FUNCTION_BLOCK FB_SignalHandlingDelay EXTENDS FB_SignalHandling
VAR_INPUT
	tDelay				: TIME;			// 延迟时间
END_VAR
VAR
	bStartProcessing	: BOOL;			// 开始延迟
	fbTimerDelay		: TON;			// TON功能块
END_VAR

// =========================================================
;
// =========================================================

METHOD SetOutput
VAR_INPUT
END_VAR
// =========================================================

IF bEnableLocal AND bInput THEN
	bStartProcessing := TRUE;
END_IF

IF bStartProcessing THEN
	fbTimerDelay(	IN := TRUE,
					PT := tDelay);
ELSE
	fbTimerDelay(	IN := FALSE);
END_IF

IF fbTimerDelay.Q THEN
	bStartProcessing := FALSE;
	
	fbTimerDelay(IN := FALSE);
	
	bOut := TRUE;
ELSE
	bOut := FALSE;
END_IF
			
// =========================================================
END_METHOD

END_FUNCTION_BLOCK
